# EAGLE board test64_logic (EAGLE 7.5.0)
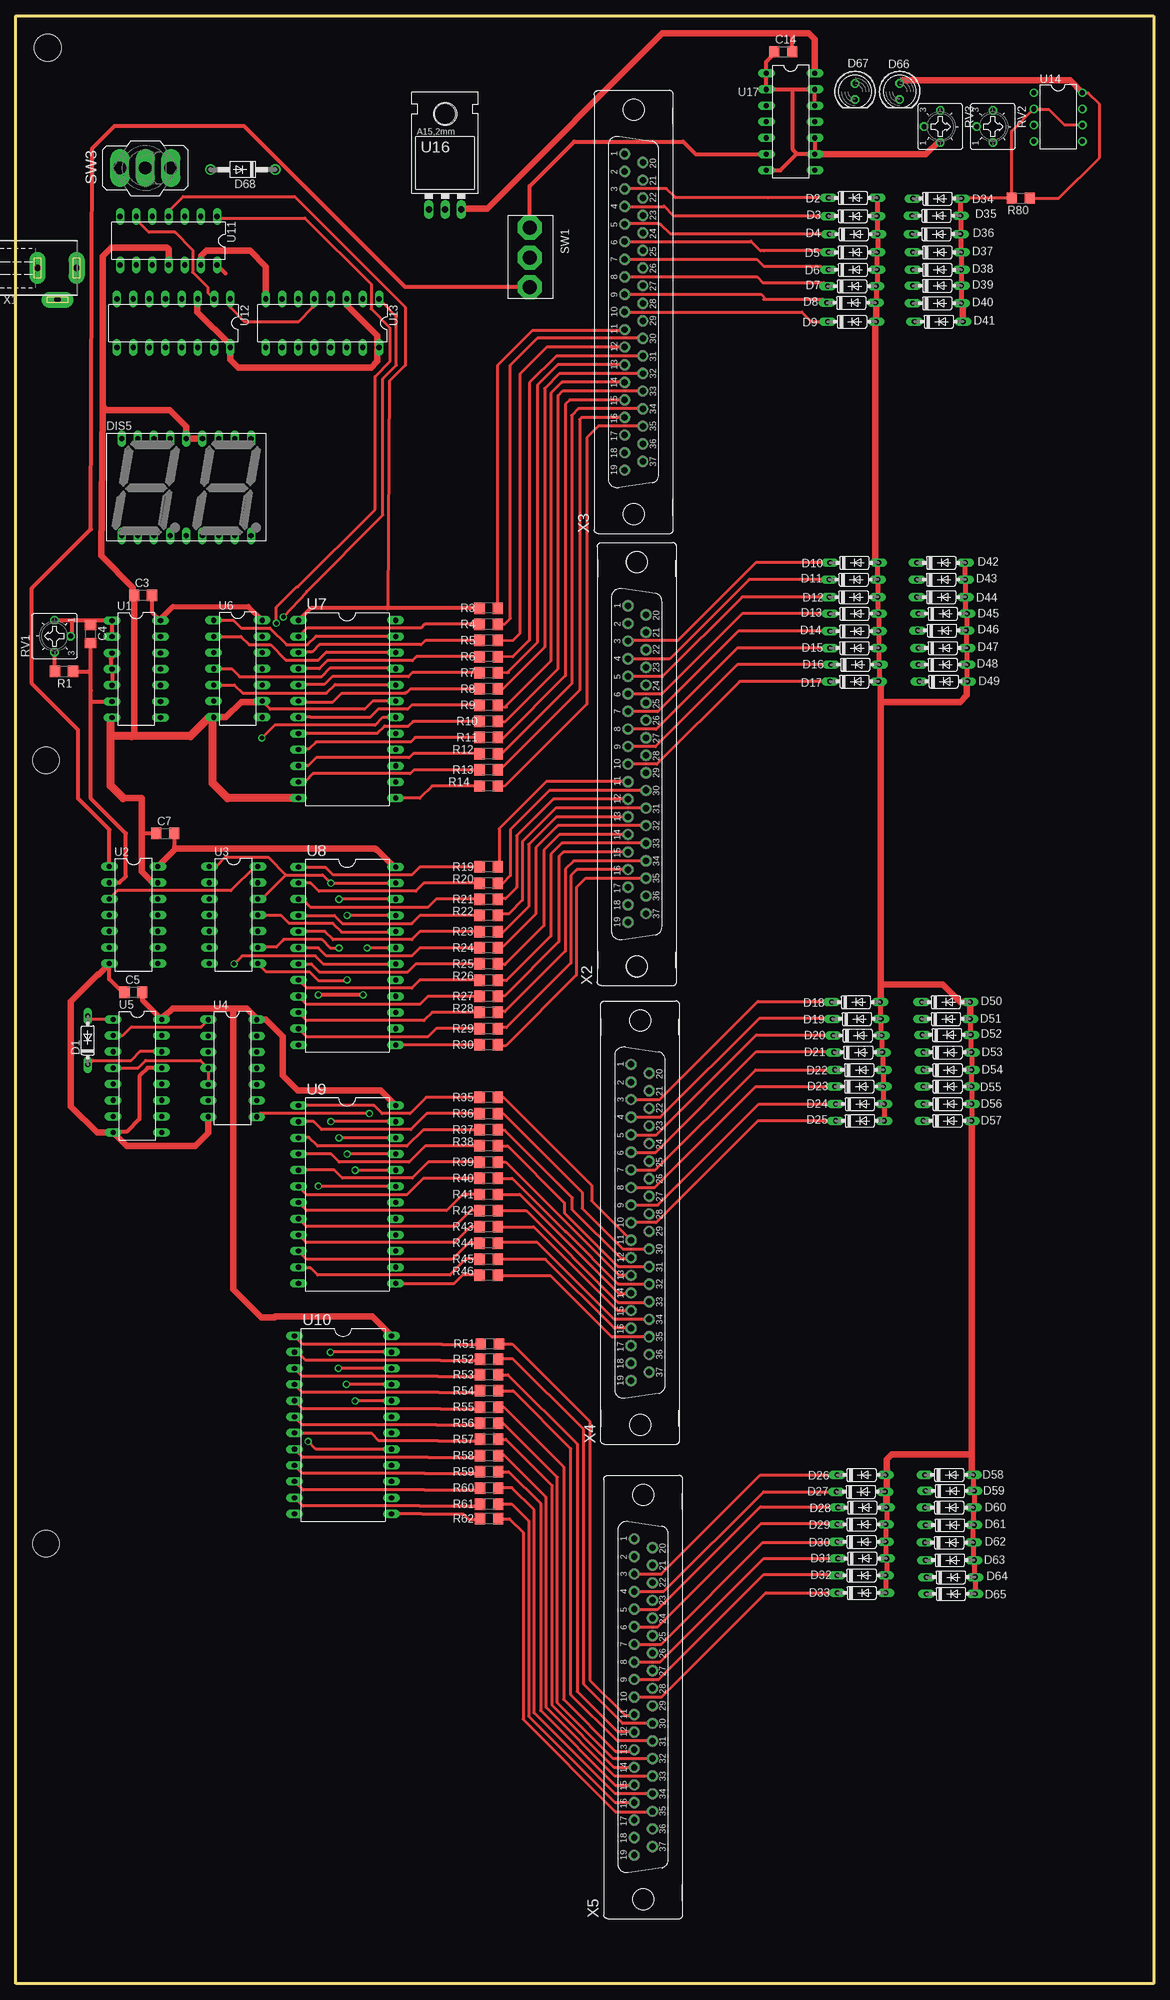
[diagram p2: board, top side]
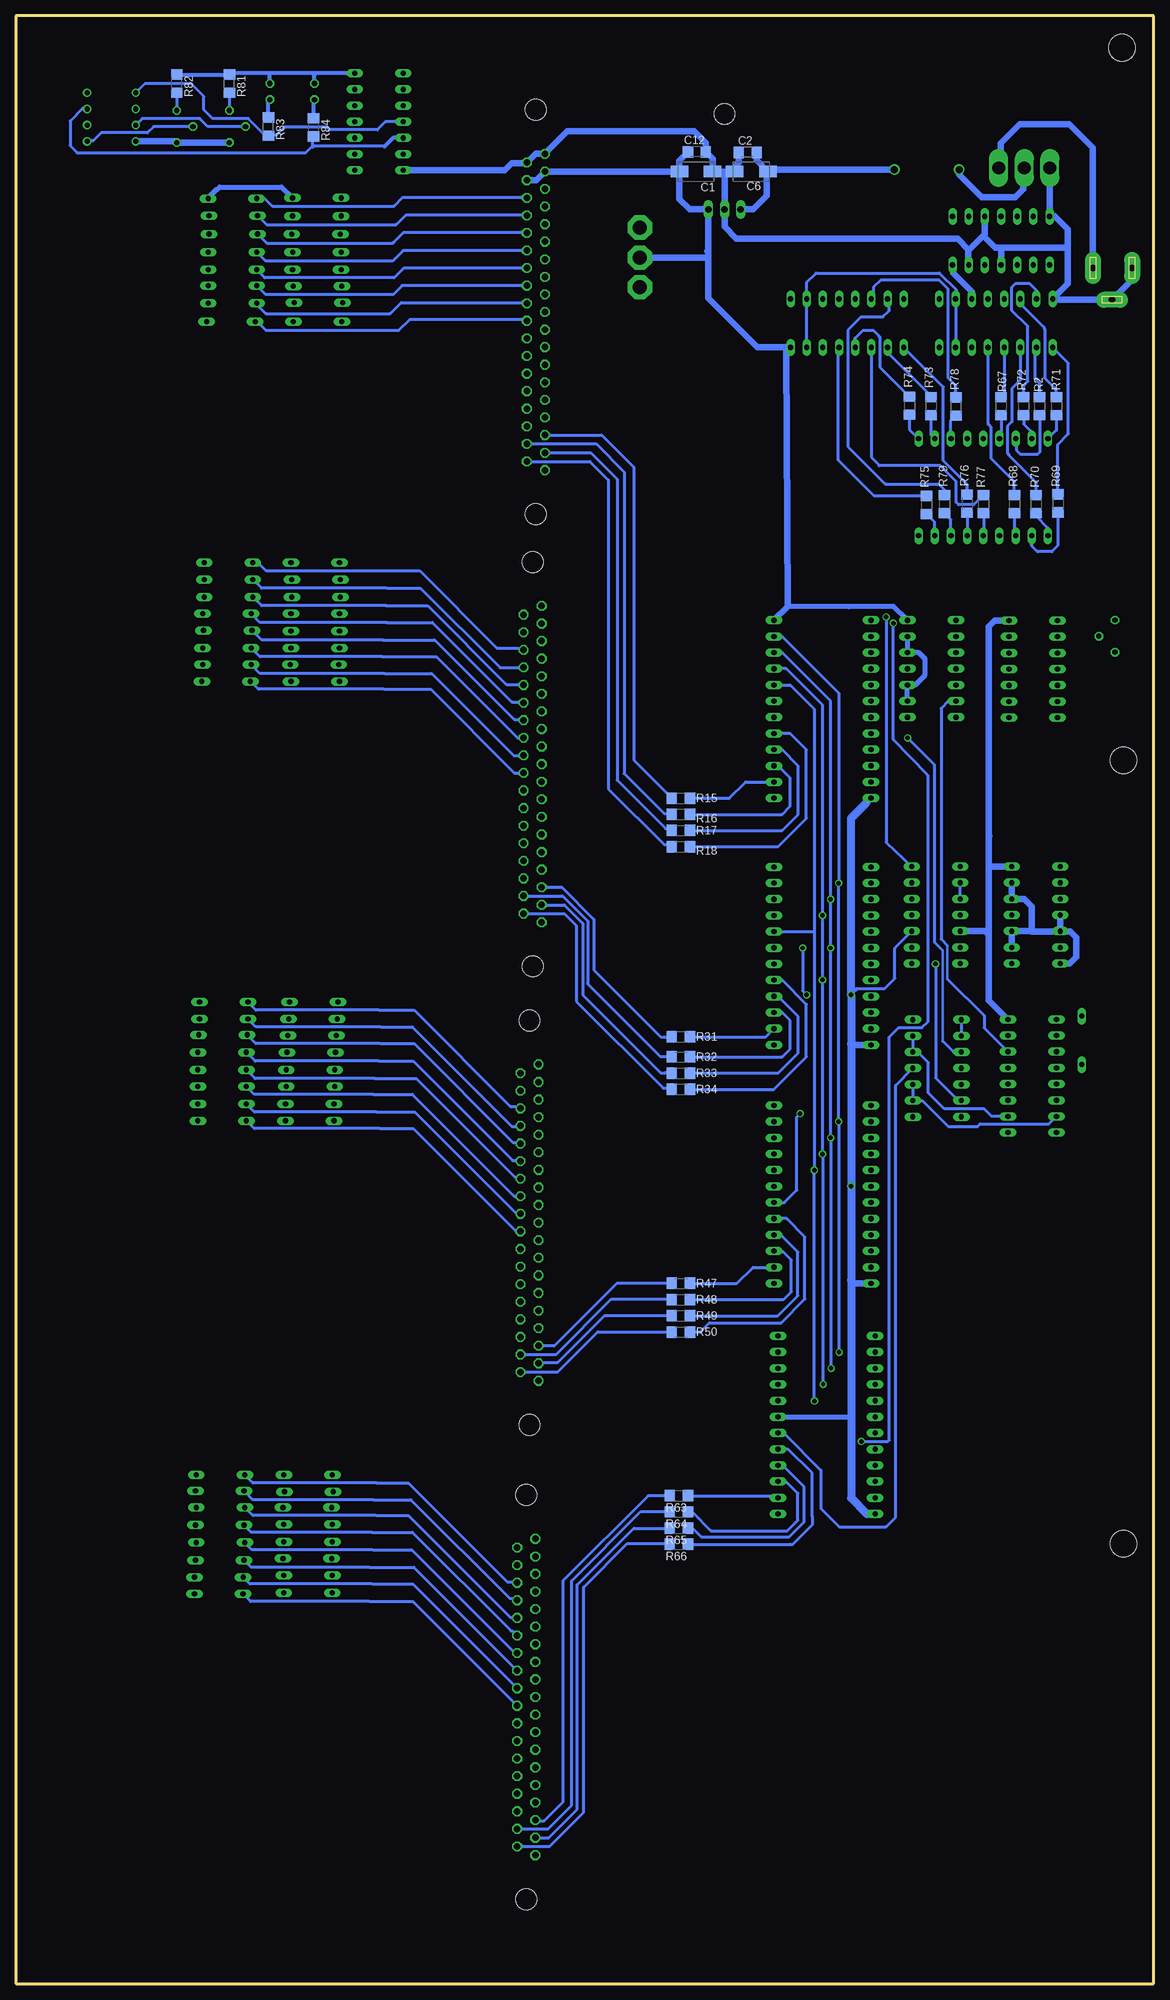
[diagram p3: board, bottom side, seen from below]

Size 178.62 x 309 mm. Coordinates in mm from the lower left corner, seen from the top.
Outline: 0,0 0,309 178.62,309 178.62,0 0,0
Copper layers (1*16): Top 0.035mm / dielectric 1.5mm / Bottom 0.035mm
Design rules "default *": minimum track width 10mil, minimum drill 24mil, track to track 8mil, track to pad 8mil, pad to pad 8mil, via to via 8mil, smd to smd 8mil, copper to edge 40mil, drill to drill 8mil, minimum pad ring 10mil, minimum via ring 8mil, stop-mask expansion 4mil, vias tented up to drill 0mil, thermal gap 10mil
Holes 4.2 mm at 5,304 4.75,69.12 4.75,192.12

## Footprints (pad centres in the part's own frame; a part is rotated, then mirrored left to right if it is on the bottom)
C/6032-28W = smd 2.75 x 1.8: + 2.625,0; - -2.625,0
C1206 = smd 1.6 x 1.8: 1 -1.4,0; 2 1.4,0
DO35-7 = drill 0.813 long: A 3.81,0; C -3.81,0
LED5MM = drill 0.813 octagon: A -1.27,0; K 1.27,0
DO41-10 = drill 1.118: A 5.08,0; C -5.08,0
HDSP-R = drill 0.813 long: 1 -10.16,-7.62; 2 -7.62,-7.62; 3 -5.08,-7.62; 4 -2.54,-7.62; 5 0,-7.62; 6 2.54,-7.62; 7 5.08,-7.62; 8 7.62,-7.62; 9 10.16,-7.62; 10 10.16,7.62; 11 7.62,7.62; 12 5.08,7.62; 13 2.54,7.62; 14 0,7.62; 15 -2.54,7.62; 16 -5.08,7.62; 17 -7.62,7.62; 18 -10.16,7.62
R1206 = smd 1.6 x 1.803: 1 -1.422,0; 2 1.422,0
CT6 = drill 0.813 octagon: A 2.515,0; E -2.515,0; S 0,-2.54
9077-1 = drill 2.2 pad 3.81 octagon: 1 4.7,-0.116; 2 0.06,-0.116; 3 -4.66,-0.116
320-916 = drill 2.007 long: 1 0,4.013; 2 0,0; 3 0,-4.013
DIL14 = drill 0.813 long: 1 -7.62,-3.81; 2 -5.08,-3.81; 3 -2.54,-3.81; 4 0,-3.81; 5 2.54,-3.81; 6 5.08,-3.81; 7 7.62,-3.81; 8 7.62,3.81; 9 5.08,3.81; 10 2.54,3.81; 11 0,3.81; 12 -2.54,3.81; 13 -5.08,3.81; 14 -7.62,3.81
DIL16 = drill 0.813 long: 1 -8.89,-3.81; 2 -6.35,-3.81; 3 -3.81,-3.81; 4 -1.27,-3.81; 5 1.27,-3.81; 6 3.81,-3.81; 7 6.35,-3.81; 8 8.89,-3.81; 9 8.89,3.81; 10 6.35,3.81; 11 3.81,3.81; 12 1.27,3.81; 13 -1.27,3.81; 14 -3.81,3.81; 15 -6.35,3.81; 16 -8.89,3.81
DIL24-6 = drill 0.813 long: 1 -13.97,-7.62; 2 -11.43,-7.62; 3 -8.89,-7.62; 4 -6.35,-7.62; 5 -3.81,-7.62; 6 -1.27,-7.62; 7 1.27,-7.62; 8 3.81,-7.62; 9 6.35,-7.62; 10 8.89,-7.62; 11 11.43,-7.62; 12 13.97,-7.62; 13 13.97,7.62; 14 11.43,7.62; 15 8.89,7.62; 16 6.35,7.62; 17 3.81,7.62; 18 1.27,7.62; 19 -1.27,7.62; 20 -3.81,7.62; 21 -6.35,7.62; 22 -8.89,7.62; 23 -11.43,7.62; 24 -13.97,7.62
DIL08 = drill 0.813 pad 1.27: 1 -3.81,-3.81; 2 -1.27,-3.81; 3 1.27,-3.81; 4 3.81,-3.81; 5 3.81,3.81; 6 1.27,3.81; 7 -1.27,3.81; 8 -3.81,3.81
78XXL = drill 1.016 long: GND 0,-3.81; IN -2.54,-3.81; OUT 2.54,-3.81 | hole 3.302: 0,11.176
733980-62 = drill 1 pad 2.5 long: 1 0,8.57; 2 0,2.42; 3 5,5.57
F37V = drill 1.016 octagon: 1 24.841,1.422; 2 22.073,1.422; 3 19.329,1.422; 4 16.561,1.422; 5 13.792,1.422; 6 11.049,1.422; 7 8.28,1.422; 8 5.512,1.422; 9 2.769,1.422; 10 0,1.422; 11 -2.769,1.422; 12 -5.512,1.422; 13 -8.28,1.422; 14 -11.049,1.422; 15 -13.818,1.422; 16 -16.561,1.422; 17 -19.329,1.422; 18 -22.098,1.422; 19 -24.841,1.422; 20 23.47,-1.422; 21 20.701,-1.422; 22 17.932,-1.422; 23 15.189,-1.422; 24 12.421,-1.422; 25 9.652,-1.422; 26 6.909,-1.422; 27 4.14,-1.422; 28 1.372,-1.422; 29 -1.372,-1.422; 30 -4.14,-1.422; 31 -6.909,-1.422; 32 -9.677,-1.422; 33 -12.421,-1.422; 34 -15.189,-1.422; 35 -17.958,-1.422; 36 -20.701,-1.422; 37 -23.47,-1.422 | hole 3.302: 31.75,0; -31.75,0

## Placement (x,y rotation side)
C1  [C/6032-28W]  71.86,284.54 180 bottom
C2  [C1206]  63.73,287.56 180 bottom
C3  [C1206]  19.95,218.03 0 top
C4  [C1206]  11.68,211.92 270 top
C5  [C1206]  18.45,155.7 0 top
C6  [C/6032-28W]  63.18,284.54 0 bottom
C7  [C1206]  23.45,180.62 0 top
C12  [C1206]  71.7,287.64 180 bottom
C14  [C1206]  120.48,303.38 0 top
D1  1N4148DO35-7  [DO35-7]  11.29,148.12 90 top
D2  1N4148DO35-7  [DO35-7]  131.38,280.43 0 top
D3  1N4148DO35-7  [DO35-7]  131.38,277.57 0 top
D4  1N4148DO35-7  [DO35-7]  131.51,274.73 0 top
D5  1N4148DO35-7  [DO35-7]  131.38,271.88 0 top
D6  1N4148DO35-7  [DO35-7]  131.38,269.15 0 top
D7  1N4148DO35-7  [DO35-7]  131.26,266.55 0 top
D8  1N4148DO35-7  [DO35-7]  131.13,263.95 0 top
D9  1N4148DO35-7  [DO35-7]  131.26,260.98 0 top
D10  1N4148DO35-7  [DO35-7]  131.62,223.12 0 top
D11  1N4148DO35-7  [DO35-7]  131.5,220.5 0 top
D12  1N4148DO35-7  [DO35-7]  131.5,217.75 0 top
D13  1N4148DO35-7  [DO35-7]  131.62,215.12 0 top
D14  1N4148DO35-7  [DO35-7]  131.62,212.38 0 top
D15  1N4148DO35-7  [DO35-7]  131.62,209.75 0 top
D16  1N4148DO35-7  [DO35-7]  131.75,207.12 0 top
D17  1N4148DO35-7  [DO35-7]  131.62,204.5 0 top
D18  1N4148DO35-7  [DO35-7]  131.88,154.12 0 top
D19  1N4148DO35-7  [DO35-7]  132,151.5 0 top
D20  1N4148DO35-7  [DO35-7]  132.12,148.88 0 top
D21  1N4148DO35-7  [DO35-7]  132.25,146.25 0 top
D22  1N4148DO35-7  [DO35-7]  132.38,143.5 0 top
D23  1N4148DO35-7  [DO35-7]  132.38,140.88 0 top
D24  1N4148DO35-7  [DO35-7]  132.5,138.12 0 top
D25  1N4148DO35-7  [DO35-7]  132.5,135.5 0 top
D26  1N4148DO35-7  [DO35-7]  132.75,79.88 0 top
D27  1N4148DO35-7  [DO35-7]  132.64,77.25 0 top
D28  1N4148DO35-7  [DO35-7]  132.88,74.75 0 top
D29  1N4148DO35-7  [DO35-7]  132.75,72.12 0 top
D30  1N4148DO35-7  [DO35-7]  132.75,69.38 0 top
D31  1N4148DO35-7  [DO35-7]  132.88,66.75 0 top
D32  1N4148DO35-7  [DO35-7]  132.75,64.12 0 top
D33  1N4148DO35-7  [DO35-7]  132.76,61.35 0 top
D34  1N4148DO35-7  [DO35-7]  144.64,280.32 0 top
D35  1N4148DO35-7  [DO35-7]  144.5,277.62 0 top
D36  1N4148DO35-7  [DO35-7]  144.5,274.75 0 top
D37  1N4148DO35-7  [DO35-7]  144.62,271.88 0 top
D38  1N4148DO35-7  [DO35-7]  144.62,269.12 0 top
D39  1N4148DO35-7  [DO35-7]  144.62,266.62 0 top
D40  1N4148DO35-7  [DO35-7]  144.62,263.88 0 top
D41  1N4148DO35-7  [DO35-7]  144.88,261 0 top
D42  1N4148DO35-7  [DO35-7]  145.25,223.12 0 top
D43  1N4148DO35-7  [DO35-7]  145.25,220.5 0 top
D44  1N4148DO35-7  [DO35-7]  145.25,217.75 0 top
D45  1N4148DO35-7  [DO35-7]  145.5,215.12 0 top
D46  1N4148DO35-7  [DO35-7]  145.38,212.5 0 top
D47  1N4148DO35-7  [DO35-7]  145.5,209.75 0 top
D48  1N4148DO35-7  [DO35-7]  145.5,207.12 0 top
D49  1N4148DO35-7  [DO35-7]  145.62,204.5 0 top
D50  1N4148DO35-7  [DO35-7]  146,154.12 0 top
D51  1N4148DO35-7  [DO35-7]  146,151.5 0 top
D52  1N4148DO35-7  [DO35-7]  146.12,149 0 top
D53  1N4148DO35-7  [DO35-7]  146.25,146.25 0 top
D54  1N4148DO35-7  [DO35-7]  146.25,143.5 0 top
D55  1N4148DO35-7  [DO35-7]  146.25,140.88 0 top
D56  1N4148DO35-7  [DO35-7]  146.25,138.12 0 top
D57  1N4148DO35-7  [DO35-7]  146.25,135.5 0 top
D58  1N4148DO35-7  [DO35-7]  146.5,79.88 0 top
D59  1N4148DO35-7  [DO35-7]  146.62,77.38 0 top
D60  1N4148DO35-7  [DO35-7]  146.5,74.75 0 top
D61  1N4148DO35-7  [DO35-7]  146.62,72 0 top
D62  1N4148DO35-7  [DO35-7]  146.5,69.25 0 top
D63  1N4148DO35-7  [DO35-7]  146.62,66.5 0 top
D64  1N4148DO35-7  [DO35-7]  146.76,63.83 0 top
D65  1N4148DO35-7  [DO35-7]  146.78,61.2 0 top
D66  [LED5MM]  138.75,297.12 270 top
D67  [LED5MM]  131.75,297.12 270 top
D68  1N4004  [DO41-10]  35.62,284.88 180 top
DIS5  HD-K123  [HDSP-R]  26.75,235 0 top
R1  [R1206]  7.54,206.06 180 top
R2  [R1206]  17.91,247.71 90 bottom
R3  [R1206]  74.22,216 0 top
R4  [R1206]  74.22,213.46 0 top
R5  [R1206]  74.22,210.92 0 top
R6  [R1206]  74.22,208.38 0 top
R7  [R1206]  74.22,205.84 0 top
R8  [R1206]  74.22,203.3 0 top
R9  [R1206]  74.22,200.76 0 top
R10  [R1206]  74.22,198.22 0 top
R11  [R1206]  74.22,195.68 0 top
R12  [R1206]  74.22,193.14 0 top
R13  [R1206]  74.22,190.6 0 top
R14  [R1206]  74.22,188.06 0 top
R15  [R1206]  74.22,186.16 180 bottom
R16  [R1206]  74.22,183.62 180 bottom
R17  [R1206]  74.22,181.07 180 bottom
R18  [R1206]  74.22,178.53 180 bottom
R19  [R1206]  74.22,175.36 0 top
R20  [R1206]  74.22,172.82 0 top
R21  [R1206]  74.22,170.28 0 top
R22  [R1206]  74.22,167.74 0 top
R23  [R1206]  74.22,165.2 0 top
R24  [R1206]  74.22,162.66 0 top
R25  [R1206]  74.22,160.12 0 top
R26  [R1206]  74.22,157.58 0 top
R27  [R1206]  74.22,155.04 0 top
R28  [R1206]  74.22,152.5 0 top
R29  [R1206]  74.22,149.96 0 top
R30  [R1206]  74.22,147.42 0 top
R31  [R1206]  74.22,148.69 180 bottom
R32  [R1206]  74.22,145.51 180 bottom
R33  [R1206]  74.22,142.97 180 bottom
R34  [R1206]  74.22,140.44 180 bottom
R35  [R1206]  74.22,139.17 0 top
R36  [R1206]  74.22,136.62 0 top
R37  [R1206]  74.22,134.08 0 top
R38  [R1206]  74.22,131.55 0 top
R39  [R1206]  74.22,129 0 top
R40  [R1206]  74.22,126.47 0 top
R41  [R1206]  74.22,123.92 0 top
R42  [R1206]  74.22,121.39 0 top
R43  [R1206]  74.22,118.84 0 top
R44  [R1206]  74.22,116.31 0 top
R45  [R1206]  74.22,113.77 0 top
R46  [R1206]  74.22,111.22 0 top
R47  [R1206]  74.22,109.95 180 bottom
R48  [R1206]  74.22,107.41 180 bottom
R49  [R1206]  74.22,104.88 180 bottom
R50  [R1206]  74.22,102.34 180 bottom
R51  [R1206]  74.41,100.45 0 top
R52  [R1206]  74.28,98.04 0 top
R53  [R1206]  74.28,95.62 0 top
R54  [R1206]  74.28,93.08 0 top
R55  [R1206]  74.28,90.54 0 top
R56  [R1206]  74.28,88 0 top
R57  [R1206]  74.28,85.46 0 top
R58  [R1206]  74.28,82.92 0 top
R59  [R1206]  74.28,80.38 0 top
R60  [R1206]  74.28,77.84 0 top
R61  [R1206]  74.28,75.3 0 top
R62  [R1206]  74.28,73.01 0 top
R63  [R1206]  74.53,76.62 180 bottom
R64  [R1206]  74.53,74.08 180 bottom
R65  [R1206]  74.53,71.54 180 bottom
R66  [R1206]  74.53,69 180 bottom
R67  [R1206]  23.95,247.71 90 bottom
R68  [R1206]  21.88,232.33 90 bottom
R69  [R1206]  15.04,232.46 90 bottom
R70  [R1206]  18.46,232.33 90 bottom
R71  [R1206]  15.26,247.71 90 bottom
R72  [R1206]  20.43,247.71 90 bottom
R73  [R1206]  34.98,247.71 90 bottom
R74  [R1206]  38.35,247.78 90 bottom
R75  [R1206]  35.65,232.21 90 bottom
R76  [R1206]  29.27,232.41 90 bottom
R77  [R1206]  26.69,232.33 90 bottom
R78  [R1206]  31.07,247.66 90 bottom
R79  [R1206]  32.86,232.33 90 bottom
R80  [R1206]  157.75,280.38 180 top
R81  [R1206]  145.12,298.38 270 bottom
R82  [R1206]  153.38,298.38 270 bottom
R83  [R1206]  139,291.62 270 bottom
R84  [R1206]  131.88,291.5 270 bottom
RV1  [CT6]  6.07,211.6 90 top
RV2  [CT6]  153.38,291.62 270 top
RV3  [CT6]  145.12,291.62 270 top
SW1  9077-1  [9077-1]  80.78,271.11 270 top
SW3  [320-916]  20.32,285.12 90 top
U1  74AC00N  [DIL14]  18.89,206.43 270 top
U2  74AC08N  [DIL14]  18.47,167.8 270 top
U3  74HC93N  [DIL14]  34.17,167.8 270 top
U4  74AC00N  [DIL14]  34,143.75 270 top
U5  4017N  [DIL16]  19.07,142.53 270 top
U6  7413N  [DIL14]  34.84,206.47 270 top
U7  74HC154N  [DIL24-6]  51.99,200.12 270 top
U8  74HC154N  [DIL24-6]  51.99,161.39 270 top
U9  74HC154N  [DIL24-6]  51.99,123.92 270 top
U10  74HC154N  [DIL24-6]  51.35,87.73 270 top
U11  74AC74N  [DIL14]  23.96,273.7 180 top
U12  4026N  [DIL16]  24.75,260.75 180 top
U13  4026N  [DIL16]  48.12,260.75 180 top
U14  LM393N  [DIL08]  163.62,293.12 270 top
U16  [78XXL]  67.38,282.43 0 top
U17  74AC08N  [DIL14]  121.62,292.38 270 top
X1  [733980-62]  0.95,269.43 270 top
X2  [F37V]  97.5,191.5 90 top
X3  [F37V]  97,262.5 90 top
X4  [F37V]  98,119.5 90 top
X5  [F37V]  98.5,45 90 top

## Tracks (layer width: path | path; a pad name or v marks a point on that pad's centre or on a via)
1
  Top 0.5: 118.1,280.43 103.58,280.43 102.12,281.88 95.62,281.88 X3.3
  Top 0.506: D2.C 118.1,280.43
2
  Bottom 0.5: 119.34,279.12 119.25,279.12 117.88,280.5 98.49,280.5 X3.22
  Bottom 0.506: D34.C 139.57,280.32 138.38,279.12 119.34,279.12
3
  Top 0.5: 120.08,277.57 103.3,277.57 101.75,279.12 101.69,279.06 X3.4
  Top 0.506: D3.C 120.08,277.57
4
  Bottom 0.5: 119,276.25 118.88,276.25 117.38,277.75 98.48,277.75 X3.23
  Bottom 0.506: D35.C 140.62,277.62 139.25,276.25 119,276.25
5
  Top 0.5: 117.48,274.73 102.78,274.73 101.25,276.25 101.12,276.25 101,276.38 95.66,276.38 X3.5
  Top 0.506: D4.C 117.48,274.73
6
  Bottom 0.5: 119.3,273.46 117.75,275 98.5,275 X3.24
  Bottom 0.506: 119.3,273.46 119.5,273.25 139.19,273.25 D36.C
7
  Top 0.5: 117.42,272.12 116.88,272.12 115.38,273.62 115.3,273.55 X3.6
  Top 0.506: D5.C 126.62,271.88 126.38,272.12 117.42,272.12
8
  Bottom 0.5: X3.25 117.85,272.15 119.08,270.91
  Bottom 0.506: 119.08,270.91 119.5,270.5 139.44,270.5 D37.C
9
  Top 0.5: X3.7 116.3,270.78 117.46,269.62
  Top 0.506: D6.C 126.85,269.15 126.38,269.62 117.46,269.62
10
  Bottom 0.5: X3.26 117.72,269.41 118.75,268.38
  Bottom 0.506: 118.75,268.38 119.25,267.88 139.56,267.88 D38.C
11
  Top 0.5: X3.8 116.36,268.01 117.25,267.12
  Top 0.506: 117.25,267.12 126.87,267.12 D7.C
12
  Bottom 0.5: X3.27 117.98,266.64 118.79,265.84
  Bottom 0.506: 118.79,265.84 119.38,265.25 139.44,265.25 D39.C
13
  Top 0.5: X3.9 116.98,265.27 117.75,264.5
  Top 0.506: 117.38,264.5 117.75,264.5 126.77,264.5 D8.C
14
  Bottom 0.5: D40.C 140.81,263.69 139.38,262.25 119.88,262.25 118.12,264 98.55,264 X3.28
15
  Top 0.5: X3.10 123.38,262.5 124.88,261 127.42,261 D9.C
16
  Bottom 0.5: D41.C 140.75,261 139.38,259.62 118.5,259.62 116.75,261.38 98.67,261.38 X3.29
17
  Top 0.5: D10.C 116.12,223.12 103.88,210.88 96.12,210.88 X2.3
18
  Bottom 0.5: D42.C 140.62,223.12 139.38,221.88 115.25,221.88 103.12,209.75 99.24,209.75 X2.22
19
  Top 0.5: D11.C 115.12,220.5 102.62,208 96.14,208 X2.4
20
  Bottom 0.5: 120.38,219.12 115.12,219.12 102.62,206.62 98.99,206.62 X2.23
  Bottom 0.506: 120.38,219.12 140.06,219.12 D43.C
21
  Top 0.5: D12.C 114,217.75 101.5,205.25 96.12,205.25 X2.5
22
  Bottom 0.5: 120.5,216.38 114,216.38 101.62,204 99,204 X2.24
  Bottom 0.506: 120.5,216.38 140.06,216.38 D44.C
23
  Top 0.5: D13.C 114,215.12 101.38,202.5 96.13,202.5 X2.6
24
  Bottom 0.5: 120.38,213.75 113.25,213.75 100.75,201.25 99.02,201.25 X2.25
  Bottom 0.506: 120.38,213.75 140.31,213.75 D45.C
25
  Top 0.5: D14.C 113.38,212.38 100.75,199.75 96.11,199.75 X2.7
26
  Bottom 0.5: 121,211 112.88,211 100.38,198.5 99.01,198.5 X2.26
  Bottom 0.506: 121,211 140.06,211 D46.C
27
  Top 0.5: D15.C 113.25,209.75 100.5,197 X2.8
28
  Bottom 0.5: 121.12,208.38 112.62,208.38 99.88,195.62 98.94,195.62 X2.27
  Bottom 0.506: 121.12,208.38 140.31,208.38 D47.C
29
  Top 0.5: D16.C 113.25,207.12 100.38,194.25 96.1,194.25 X2.9
30
  Bottom 0.5: 120.75,205.75 113.38,205.75 100.5,192.88 X2.28
  Bottom 0.506: 120.75,205.75 140.31,205.75 D48.C
31
  Top 0.5: D17.C 113.62,204.5 100.62,191.5 X2.10
32
  Bottom 0.5: 120.88,203.25 113.5,203.25 100.38,190.12 X2.29
  Bottom 0.506: 120.88,203.25 140.56,203.25 D49.C
33
  Top 0.5: X4.3 101.08,138.83 116.5,154.25 127.94,154.25 D18.C
34
  Bottom 0.5: 121.62,152.88 116.12,152.88 101,137.75 99.74,137.75 X4.22
  Bottom 0.506: 121.62,152.88 140.94,152.88 D50.C
35
  Top 0.5: X4.4 101.19,136.06 116.75,151.62 128.06,151.62 D19.C
  Top 0.506: 127.25,151.38 128.06,151.38 D19.C
36
  Bottom 0.5: 121.38,150.25 116.38,150.25 100.75,134.62 99.49,134.62 X4.23
  Bottom 0.506: 121.38,150.25 140.94,150.25 D51.C
37
  Top 0.5: X4.5 100.54,133.29 116.25,149 127.5,149
  Top 0.506: 127.5,149 128.19,149 D20.C
38
  Bottom 0.5: 121.5,147.62 116.12,147.62 100.62,132.12 99.63,132.12 X4.24
  Bottom 0.506: 121.5,147.62 140.94,147.62 D52.C
39
  Top 0.5: X4.6 100.42,130.55 116.25,146.38 127.75,146.38 127.88,146.25
  Top 0.506: D21.C 127.88,146.25 127.62,146.25
40
  Bottom 0.5: 121.62,144.88 116.25,144.88 100.62,129.25 99.52,129.25 X4.25
  Bottom 0.506: 121.62,144.88 141.06,144.88 D53.C
41
  Top 0.5: X4.7 100.41,127.78 116.12,143.5 D22.C
42
  Bottom 0.5: 122.25,142.12 115.75,142.12 100.25,126.62 99.64,126.62 X4.26
  Bottom 0.506: 122.25,142.12 141.06,142.12 D54.C
43
  Top 0.5: X4.8 100.26,125.01 116.12,140.88 D23.C
44
  Bottom 0.5: 122.5,139.62 116.38,139.62 100.38,123.62 99.44,123.62 X4.27
  Bottom 0.506: 122.5,139.62 141.19,139.62 D55.C
45
  Top 0.5: X4.9 100.77,122.27 116.62,138.12 D24.C
46
  Bottom 0.5: 122,136.88 116,136.88 100.12,121 99.55,121 X4.28
  Bottom 0.506: 122,136.88 141.19,136.88 D56.C
47
  Top 0.5: D25.C 116.5,135.5 100.5,119.5 X4.10
48
  Bottom 0.5: 121.5,134.25 116.25,134.25 100,118 99.55,118 X4.29
  Bottom 0.506: 121.5,134.25 141.19,134.25 D57.C
49
  Top 0.5: X5.3 101.33,64.33 116.88,79.88 D26.C
50
  Bottom 0.5: 122,78.62 117,78.62 101.5,63.12 100.11,63.12 X5.22
  Bottom 0.506: 122,78.62 141.44,78.62 D58.C
51
  Top 0.5: X5.4 101.69,61.56 117.38,77.25 D27.C
52
  Bottom 0.5: 122.5,76 116.62,76 101.12,60.5 100.23,60.5 X5.23
  Bottom 0.506: 122.5,76 141.44,76 D59.C
53
  Top 0.5: X5.5 100.79,58.79 116.88,74.88 128.94,74.88 D28.C
54
  Bottom 0.5: 122.12,73.5 117,73.5 101,57.5 100,57.5 X5.24
  Bottom 0.506: 122.12,73.5 141.44,73.5 D60.C
55
  Top 0.5: X5.6 100.8,56.05 117,72.25 128.81,72.25 D29.C
56
  Bottom 0.5: 122.75,70.88 116.38,70.88 100.88,55.38 100.64,55.38 X5.25
  Bottom 0.506: 122.75,70.88 141.69,70.88 D61.C
57
  Top 0.5: X5.7 101.28,53.28 117.25,69.25 128.38,69.25 128.5,69.12 128.69,69.12 D30.C
58
  Bottom 0.5: 122.62,68.12 116.5,68.12 100.5,52.12 100.14,52.12 X5.26
  Bottom 0.506: 122.62,68.12 141.56,68.12 D62.C
59
  Top 0.5: X5.8 101.14,50.51 117.38,66.75 D31.C
60
  Bottom 0.5: 123.12,65.38 116.16,65.38 X5.27
  Bottom 0.506: 123.12,65.38 141.69,65.38 D63.C
61
  Top 0.5: X5.9 100.89,47.77 117.38,64.25 128.81,64.25 D32.C
62
  Bottom 0.5: 122.75,62.75 116.3,62.75 X5.28
  Bottom 0.506: 122.75,62.75 141.88,62.75 D64.C
63
  Top 0.5: X5.10 101.38,45 117.75,61.38 128.93,61.38 D33.C
64
  Bottom 0.5: 123.12,60 116.29,60 X5.29
  Bottom 0.506: 123.12,60 141.76,60 D65.C
+5V
  Top 0.5: R80.1 163.75,280.38 170.12,286.75 170.12,295.12 168.38,296.88 167.5,296.88 U14.8
  Top 0.51: 44.15,104.9 44,104.75
  Top 0.61: C7.2 24.86,178.5 25.11,178.25 | 32.88,268.59 U11.14 | C3.2 21.36,215.4 U1.14 | C14.2 121.88,305.75 122.38,306.25
  Top 0.813: U1.14 22.7,214.33 24.62,216.25 36.5,216.25 U6.14 | C5.2 19.86,154.44 U5.16
  Top 1.016: U2.14 25.11,178.25 56.38,178.25 56.5,178.12 56.62,178.12 59.39,175.36 U8.24 | U13.3 51.94,263.56 56.75,258.75 56.75,257.21 U13.16 56.75,256.68 56.75,254.75 55.75,253.75 34.88,253.75 33.64,254.99 U12.16 33.64,257.36 28.5,262.5 28.5,264.5 U12.3 | 33.88,153.12 36.25,153.12 37.81,151.56 U4.14 39.25,151.38 41.88,148.75 41.88,142.62 44.25,140.25 57.26,140.25 U9.24 | 33.88,153.12 24.59,153.12 23.38,151.92 | 33.88,153.12 34.12,152.88 34.12,109 38.5,104.62 40.62,104.62 40.75,104.75 44,104.75 55.92,104.75 U10.24 | U16.OUT 70.05,278.75 74,278.75 101.5,306.25 122.38,306.25 124.5,306.25 125.44,305.31 U17.14 | U14.8 165.5,298.88 139.23,298.88 D66.A
  Top 1.27: 23.38,151.92 U5.16
  Bottom 0.61: U17.14 132,300 | 132,300 138.62,300 | 138.62,300 144.93,300 R81.1 R82.1 | D66.A 138.75,299.87 138.62,300 | D67.A 131.75,299.75 132,300
  Bottom 0.813: U6.14 38.72,214.09 40.88,216.25 47.88,216.25 | 47.88,216.25 57.45,216.25 | 47.84,216.21 47.88,216.25
  Bottom 1.016: U12.3 28.56,265.69 31.5,268.62 31.5,269.81 U11.14 | U1.14 24.95,214.04 25.88,213.12 25.88,180.25 | 25.88,180.25 25.88,175.5 | 25.88,175.5 25.88,164.75 | 25.88,164.75 25.88,154.42 U5.16 | U2.14 25.8,175.42 25.88,175.5 | U3.5 26.39,165.26 25.88,164.75 | 25.8,180.18 25.88,180.25 | C1.+ 74.48,286.26 C12.2 | 69.92,272.25 U16.OUT 72.87,278.62 74.5,280.25 C1.+ | 69.92,272.25 69.92,271 | 69.92,271 69.92,264.66 62.25,257 57.08,257 U13.16 57.7,256.25 57.45,216.25 U7.24 | 70.11,272.05 69.92,272.25 | SW1.2 69.97,271.05 69.92,271 | C1.+ 74.51,284.57 X3.2 96.95,283.2 X3.21
A  (via drill 0.7)
  Top 0.5: v49.45,172.82 U8.23 | U9.23 v49.45,135.36 | U3.1 31.42,175.42 32.88,176.88 39.62,176.88 42.38,174.12
  Top 0.506: U6.1 34.16,214.09 35.38,212.88 39.88,212.88 42.5,210.25 45.75,210.25 47.12,211.62 59.54,211.62 U7.23 | v49.45,172.82 48.15,174.12 42.38,174.12 38.59,170.34 U3.12 | U10.23 49.41,99.16 v49.38,99.12
  Bottom 0.5: U7.23 58.34,211.56 49.45,202.66 v49.45,172.82 v49.45,135.36
  Bottom 0.506: v49.38,99.12 49.38,135.28 v49.45,135.36
A1
  Bottom 0.5: R2.1 17.91,240.47 18.25,240.12 20.88,240.12 21.5,240.75 21.5,242.45 DIS5.16
A2
  Bottom 0.5: R73.1 34.98,243.22 DIS5.11
B  (via drill 0.7)
  Top 0.5: U8.22 v50.72,170.28 | U9.22 v50.72,132.81
  Top 0.506: U6.2 35.32,211.56 36.62,210.25 40,210.25 42.38,207.88 47.5,207.88 48.75,209.12 59.5,209.12 U7.22 | v50.72,162.62 49.38,162.62 48,164 42,164 42,163.88 40.88,162.75 38.01,162.75 U3.9 | U10.22 v50.63,96.62 v50.62,96.62
  Bottom 0.5: U7.22 58.34,209.01 50.72,201.4 v50.72,170.28 50.72,164.88 | v50.72,132.81 v50.72,162.62
  Bottom 0.506: v50.72,162.62 50.72,164.88 | v50.62,96.62 50.62,132.72 v50.72,132.81
B1
  Bottom 0.5: R67.1 23.95,242.88 DIS5.15
B2
  Bottom 0.5: R74.1 38.35,244.06 DIS5.10
C  (via drill 0.7)
  Top 0.5: U8.21 v51.99,167.74 | U9.21 v51.99,130.28
  Top 0.506: U6.4 33.9,206.47 35.12,205.25 48,205.25 49.38,206.62 59.46,206.62 U7.21 59.59,206.5 | v51.99,157.62 51.87,157.5 47.5,157.5 46.12,158.88 39.28,158.88 U3.8 | U10.21 51.92,94.08 v51.88,94.12
  Bottom 0.5: U7.21 57.7,206.47 51.99,200.76 v51.99,167.74 51.99,160.75 | v51.99,130.28 v51.99,157.62 | 51.99,158.62 51.99,160
  Bottom 0.506: 51.99,160 51.99,160.75 | v51.99,157.62 51.99,158.62 | v51.88,94.12 51.88,130.16 v51.99,130.28
C1
  Bottom 0.5: R68.1 21.88,227.59 DIS5.3
C2
  Bottom 0.5: DIS5.8 34.37,229.51 R75.1
CL  (via drill 0.7)
  Top 0.5: U3.14 37.55,175.42 33.75,171.62 15.95,171.62 U2.3 | U13.1 57.02,264.49 59.75,261.75 59.75,254.12 57.62,252 57.62,230.62 45.62,218.62 45.62,218.5 v42,214.62
  Bottom 0.5: 37.17,175.42 U3.14 42,179.19 v42,214.62
D  (via drill 0.7)
  Top 0.5: v53.26,127.73 U9.20
  Top 0.506: U6.5 34.31,203.94 35.62,202.62 48.75,202.62 50.12,204 59.55,204 U7.20 | 59.56,165.25 U8.20 59.53,165.12 51.12,165.12 49.75,166.5 42.88,166.5 41.62,167.75 38.03,167.75 U3.11 | U10.20 53.29,91.54 v53.25,91.5
  Bottom 0.5: U7.20 57.07,203.94 53.26,200.12 53.26,165.2 | 53.26,165.2 v53.26,127.73 | U8.20 53.26,165.2
  Bottom 0.506: v53.25,91.5 v53.25,127.72 v53.26,127.73
D1
  Bottom 0.5: R69.1 15.04,225.83 16,224.88 18.25,224.88 19.12,225.75 DIS5.2
D2
  Bottom 0.5: R76.1 29.27,227.4 DIS5.6
E1
  Bottom 0.5: DIS5.1 16.59,228.59 18.46,230.47 R70.1
E2
  Bottom 0.5: R77.1 26.69,227.44 DIS5.5
F1
  Bottom 0.5: R71.1 15.26,243.95 DIS5.18
F2
  Bottom 0.5: DIS5.12 31.83,245.47 R78.1
G1
  Bottom 0.5: R72.1 20.43,244.93 19.25,243.75 19.25,242.74 DIS5.17
G2
  Bottom 0.5: DIS5.7 31.83,229.88 R79.1
GND  (via drill 0.7)
  Top 0.5: U7.19 56.02,201.4 54.75,200.12 39.92,200.12 U6.9 | U8.19 55.16,162.66 v55.12,162.62 | U9.19 47.55,125.19 v47.5,125.25
  Top 0.61: v54.5,155.25 v47.5,155.25 | C5.1 16.68,155.7 14.62,157.75 14.62,160.14 U2.7 | U5.13 20.68,143.8 19.38,142.5 19.38,135.75 17.38,133.75 15.37,133.75 U5.8 | C7.1 20.13,180.62 19.75,181 | 39.02,268.59 39.23,268.38 | C14.1 119.08,303.08 117.75,301.75 117.75,300.06 U17.1 U17.2 121.88,297.46 | 121.88,297.46 U17.13 U17.12 | 122.62,287.38 122.7,287.29 U17.9 U17.10 | 122.62,287.38 122,288 122,297.33 121.88,297.46 | U17.7 120,284.75 122.62,287.38
  Top 1.016: U13.8 39.23,268.38 39.23,269.64 36.75,272.12 29.88,272.12 29.12,271.38 29.12,269.98 U11.13 | DIS5.13 DIS5.14 26.75,244.5 24.12,247.12 14.12,247.12 13.62,247.62 | U11.11 23.96,272.38 23.71,272.62 15,272.62 13.62,271.25 13.62,247.62 | 16.84,186.16 19.72,186.16 19.75,186.12 19.75,181 19.75,174.62 21.62,172.75 22.15,172.75 U2.13 | U6.7 32.98,198.85 35.38,201.25 38.51,201.25 U6.9 | 13.62,247.62 13.38,224.25 18.38,219.25 18.38,218.21 C3.1 18.55,196.31 18.12,195.88 | U2.7 12.98,158.5 12.88,158.5 8.62,154.25 8.62,137.75 12.73,133.64 U5.8 17.4,131.5 28.12,131.5 30.19,133.56 U4.7 | RV3.A 144.74,289.11 142.88,287.25 125.48,287.25 U17.9
  Top 1.27: 16.84,186.16 14.88,188.12 14.88,195.75 | 14.88,195.75 14.88,198.59 U1.7 | 14.88,195.75 15,195.88 18.12,195.88 27.38,195.88 30.36,198.85 U6.7 30.88,198.69 30.88,188.5 33.22,186.16 U7.12
  Bottom 0.5: v55.12,162.62 55.12,155.88 v54.5,155.25 | U3.10 40.62,162.62 40.62,157.88 42.25,156.25 46.75,156.25 46.75,156 v47.5,155.25
  Bottom 0.813: U6.9 U6.10 37.44,203.94 35.88,205.5 35.88,208 36.88,209 38.64,209 U6.12 U6.13 | 47.3,147.42 47.5,147.62 | 46.95,109.95 47.5,110.5 | U10.19 47.5,89
  Bottom 1.016: U11.3 26.5,274.75 26.75,274.5 | 26.75,274.5 29,272.25 | 29,272.25 29.12,272.12 29.12,269.98 U11.13 | 23.96,271.34 U11.11 23.96,272.46 24.12,272.62 | 13.5,272.38 13.5,275.5 15.51,277.51 U11.7 16.3,277.55 SW3.1 | 13.5,272.38 13.5,266.92 U12.8 15.73,264.43 X1.3 3.38,267.58 X1.2 | 24.12,272.62 13.75,272.62 13.5,272.38 | 24.12,272.62 24.88,272.62 26.75,274.5 | U2.13 U2.12 20.34,170.34 19.12,169.12 19.12,165.25 | 19.12,165.25 15.25,165.25 | 15.25,165.25 U2.5 13.12,165.25 12.12,164.25 12.12,161.25 13.2,160.18 U2.7 | 19.12,165.25 19.14,165.26 U2.10 U2.9 | U2.4 14.66,165.84 15.25,165.25 | 29,272.25 30.75,274 65.5,274 67.38,275.88 U16.GND 67.38,284.42 67.5,284.54 | C6.- 66.5,284.54 | 66.5,284.54 67.5,284.54 | 67.5,284.54 C1.- 69.23,286.56 C12.1 70.31,289.06 72.12,290.88 92.04,290.88 X3.1 97.05,287.34 X3.20 98.52,285.88 100.75,285.88 101.87,284.75 U17.7 | C2.2 65.12,285.92 66.5,284.54 | 45.2,185.32 U7.12 | U14.4 153.58,289.31 RV2.A RV3.A | 46.95,109.95 U9.12 | 47.3,147.42 U8.12 | 45.01,73.76 U10.12
  Bottom 1.27: 45.01,73.76 47.5,76.25 47.5,89 47.5,110.5 v47.5,125.25 47.5,147.62 v47.5,155.25 47.5,183.03 45.2,185.32
L1
  Top 0.5: R3.2 75.64,254.14 81.12,259.62 95.47,259.62 X3.11
L2
  Top 0.5: R4.2 76.71,213.46 77.62,214.38 77.62,254.12 81.86,258.36 X3.30
L3
  Top 0.406: 78.03,210.92 R5.2
  Top 0.5: X3.12 83.36,256.99 79.12,252.75 79.12,212.02 78.03,210.92
L4
  Top 0.406: R6.2 78.03,208.38
  Top 0.5: X3.31 84.84,255.59 80.62,251.38 80.62,210.98 78.03,208.38
L5
  Top 0.406: R7.2 77.12,205.84 77.39,205.84
  Top 0.5: X3.13 85.09,254.22 81.88,251 81.88,210.59 77.12,205.84
L6
  Top 0.406: R8.2 76.44,203.3
  Top 0.5: X3.32 85.32,252.82 83,250.5 83,209.86 76.44,203.3
L7
  Top 0.406: R9.2 75.95,200.44 76.75,200.44 77.07,200.44
  Top 0.5: X3.14 85.7,251.45 84,249.75 84,207.69 76.75,200.44
L8
  Top 0.406: R10.2 76.12,198.22
  Top 0.5: 76.12,198.22 76.84,198.22 85.12,206.5 85.12,249.38 85.88,250.12 98.38,250.12 X3.33
L9
  Top 0.406: R11.2 76.12,195.68 76.34,195.46
  Top 0.5: X3.15 86.93,248.68 86.25,248 86.25,205.38 76.34,195.46
L10
  Top 0.406: R12.2 75.64,192.99
  Top 0.5: X3.34 88.31,247.31 87.25,246.25 87.25,204.12 76.25,193.12 75.65,193.12 R12.2
L11
  Top 0.406: R13.2 76.12,190.6
  Top 0.5: X3.16 88.81,245.94 88.5,245.62 88.5,203.12 76.25,190.88 75.91,190.88 R13.2
L12
  Top 0.406: R14.2 76.75,188.06
  Top 0.5: X3.35 91.42,244.54 89.62,242.75 89.62,200.93 76.75,188.06
L13
  Bottom 0.5: X3.17 86.67,243.17 81.62,238.12 81.62,192.14 R15.2
L14
  Bottom 0.5: X3.36 87.55,241.8 83.12,237.38 83.12,190 76.88,183.75 75.25,183.75 75.12,183.62 75.63,183.62 R16.2
L15
  Bottom 0.5: X3.18 88.4,240.4 84.25,236.25 84.25,189 76.62,181.38 75.94,181.38 R17.2
L16
  Bottom 0.5: X3.37 88.53,239.03 85.62,236.12 85.62,187.62 76.88,178.88 75.98,178.88 R18.2
L17
  Top 0.5: X2.11 83.23,188.73 75.88,181.38 75.88,175.6 R19.2
L18
  Top 0.5: X2.30 83.73,187.36 77.62,181.25 77.62,174 76.25,172.62 75.83,172.62 R20.2
L19
  Top 0.5: X2.12 84.36,185.99 78.62,180.25 78.62,172.12 76.88,170.38 75.73,170.38 R21.2
L20
  Top 0.5: 75.64,167.89 R22.2 76.25,167.75 76.5,168 77.38,168 79.5,170.12 79.5,179.38 84.72,184.59 X2.31
L21
  Top 0.5: X2.13 84.84,183.22 80.5,178.88 80.5,169.12 76.5,165.12 75.71,165.12 R23.2
L22
  Top 0.5: X2.32 85.07,181.82 81.62,178.38 81.62,168 76.5,162.88 75.85,162.88 R24.2
L23
  Top 0.5: X2.14 85.33,180.45 82.88,178 82.88,166.12 76.75,160 75.76,160 R25.2
L24
  Top 0.5: X2.33 85.7,179.08 84,177.38 84,164.5 77,157.5 75.72,157.5 R26.2
L25
  Top 0.5: X2.15 85.93,177.68 85.25,177 85.25,163.62 76.75,155.12 75.72,155.12 R27.2
L26
  Top 0.5: X2.34 87.56,176.31 86.25,175 86.25,162.12 76.75,152.62 76.25,152.62 75.88,153 75.88,152.74 R28.2
L27
  Top 0.5: X2.16 88.06,174.94 87.12,174 87.12,160.25 77,150.12 75.8,150.12 R29.2
L28
  Top 0.5: X2.35 89.42,173.54 88,172.12 88,158.38 76.88,147.25 75.81,147.25 R30.2
L29
  Bottom 0.5: R31.2 77.39,148.69 87.88,159.18 87.88,167.12 92.92,172.17 X2.17
L30
  Bottom 0.5: R32.2 77.39,145.51 88.88,157 88.88,166.88 92.8,170.8 X2.36
L31
  Bottom 0.5: R33.2 76.75,142.97 76.78,143 77.38,143 89.62,155.25 89.62,166.5 92.53,169.4 X2.18
L32
  Bottom 0.5: 76.12,140.44 R34.2 75.83,140.62 77,140.62 90.62,154.25 90.62,166.12 92.53,168.03 X2.37
L33
  Top 0.5: X4.11 90.38,122.93 90.38,125.38 76.58,139.17 R35.2
L34
  Top 0.5: X4.30 99.41,115.38 95.25,115.38 88.88,121.75 88.88,124.25 76.5,136.62 R36.2
L35
  Top 0.5: X4.12 96.46,113.88 95,113.88 87.38,121.5 87.38,123.38 76.75,134 75.72,134 R37.2
L36
  Top 0.5: X4.31 99.39,112.62 94.5,112.62 86.12,121 86.12,122.62 77.2,131.55 R38.2
L37
  Top 0.5: X4.13 96.55,111.25 94.62,111.25 76.87,129 R39.2
L38
  Top 0.5: X4.32 99.37,109.88 94.5,109.88 86.38,118 86.25,118.12 77.91,126.47 R40.2
L39
  Top 0.5: X4.14 96.5,108.38 94.62,108.38 79.08,123.92 R41.2
L40
  Top 0.5: X4.33 99.34,107 94.5,107 80.11,121.39 R42.2
L41
  Top 0.5: X4.15 96.51,105.75 94.38,105.75 81.28,118.84 R43.2
L42
  Top 0.5: 76.12,116.31 R44.2 75.71,116.38 81.88,116.38 93.94,104.31 X4.34
L43
  Top 0.5: R45.2 76.25,113.77 | 76.25,113.77 76.44,113.77 | X4.16 93.94,102.94 83.12,113.75 76.27,113.75 76.25,113.77
L44
  Top 0.5: R46.2 76.44,111.22 76.54,111.12 84,111.12 93.58,101.54 X4.35
L45
  Bottom 0.5: 75.64,110.42 R47.2 84.3,109.95 94.12,100.12 96.53,100.12 X4.17
L46
  Bottom 0.5: X4.36 93.83,98.8 85.12,107.5 75.72,107.5 R48.2
L47
  Bottom 0.5: R49.2 86.25,104.88 93.62,97.5 96.48,97.5 X4.18
L48
  Bottom 0.5: 76.12,102.34 R50.2 75.68,102.38 87.25,102.38 93.59,96.03 X4.37
L49
  Top 0.5: R51.2 77.92,100.45 90.12,88.25 90.12,47.62 95.62,42.12 96.97,42.12 X5.11
L50
  Top 0.5: X5.30 95.27,40.86 89.12,47 89.12,87 78,98.12 75.79,98.12 R52.2
L51
  Top 0.5: X5.12 96.94,39.62 94.38,39.62 88.12,45.88 88.12,84.75 77.25,95.62 R53.2
L52
  Top 0.5: X5.31 94.41,38.09 87.12,45.38 87.12,84 78.04,93.08 R54.2 75.75,93.12
L53
  Top 0.5: X5.13 96.86,36.5 94.12,36.5 86,44.62 86,81.12 76.58,90.54 R55.2
L54
  Top 0.5: X5.32 93.8,35.32 85,44.12 85,79.5 76.5,88 R56.2
L55
  Top 0.5: X5.14 97.03,34 93.88,34 84.12,43.75 84.12,78.25 76.91,85.46 R57.2
L56
  Top 0.5: X5.33 94.05,32.58 83.25,43.38 83.25,76.38 76.62,83 75.78,83 R58.2
L57
  Top 0.5: X5.15 97.02,31.12 94.12,31.12 82.38,42.88 82.38,75.38 77.37,80.38 R59.2
L58
  Top 0.5: X5.34 94.06,29.81 81.38,42.5 81.38,74.38 77.88,77.88 75.74,77.88 R60.2
L59
  Top 0.5: R61.2 77.82,75.3 80.5,72.62 80.5,42 94,28.5 97.02,28.5 X5.16
L60
  Top 0.5: R62.2 77.49,73.01 79.62,70.88 79.62,41.5 94.12,27 99.88,27 X5.35
L61
  Bottom 0.5: R63.2 79.38,76.62 92.75,63.25 92.75,28.5 95.75,25.5 96.91,25.5 X5.17
L62
  Bottom 0.5: X5.36 95.08,24.3 91.38,28 91.38,63.25 80.5,74.12 76,74.12 R64.2
L63
  Bottom 0.5: X5.18 94.97,22.9 90.5,27.38 90.5,62.62 81.62,71.5 75.99,71.5 R65.2
L64
  Bottom 0.5: X5.37 94.84,21.53 89.5,26.88 89.5,62.25 82.62,69.12 76.08,69.12 R66.2
MR
  Bottom 0.5: U3.3 U3.2
N$1
  Top 0.61: U1.3 15.09,208.21 14.88,208 14.88,206.63 U1.4 U1.5
N$2
  Top 0.61: RV1.A 8.88,214.12 | 8.88,214.12 11.62,214.12 | 11.62,214.12 15.09,214.12 U1.1 U1.2 | RV1.S 8.88,211.6 8.88,214.12 | C4.1 11.62,213.32 11.62,214.12
N$3
  Top 0.5: 14.99,201.25 14.12,201.25
  Top 0.61: C4.2 11.68,205.75 | 11.68,205.75 11.68,203.19 11.75,203.12 11.75,201.38 | U1.6 14.99,201.25 11.88,201.25 11.75,201.38 | R1.1 11.37,206.06 11.68,205.75 | U2.2 16.25,172.88 17.25,173.88 17.25,180.62 11.75,186.12 11.75,201.38
N$5
  Top 0.61: R1.2 6.12,209.03 RV1.E
N$6
  Top 0.5: U11.6 18.88,277 20.88,275 25,275 27.75,272.25 27.75,268.75 30.12,266.38 30.12,265.53 U12.2
  Bottom 0.5: U12.15 U12.2 31,264.66 31,266 33.62,268.62 53,268.62 54.48,267.15 U13.2 U13.15
N$7
  Top 0.506: R4.1 64.21,213.46 63.62,212.88 45.69,212.88 U7.2
N$8
  Top 0.506: R5.1 64.3,210.92 63.62,210.25 47.62,210.25 46.5,209.12 44.48,209.12 U7.3
N$9
  Top 0.506: R6.1 62.88,208.38 62.25,207.75 48.88,207.75 47.62,206.5 44.4,206.5 U7.4
N$10
  Top 0.506: R7.1 62.22,205.84 61.62,205.25 49.62,205.25 48.38,204 44.44,204 U7.5
N$11
  Top 0.506: R8.1 61.92,203.3 61.38,202.75 61.25,202.75 61.12,202.62 51.12,202.62 49.75,201.25 44.52,201.25 U7.6
N$12
  Top 0.5: 46.25,198.88 55.62,198.88 56.88,200.12
  Top 0.506: R9.1 62.13,200.76 61.5,200.12 56.88,200.12 | 46.25,198.88 44.39,198.88 U7.7
N$13
  Top 0.5: 47.38,196.38 56.75,196.38 57.88,197.5
  Top 0.506: R10.1 62.34,198.22 61.62,197.5 57.88,197.5 | U7.8 44.43,196.38 47.38,196.38
N$14
  Top 0.506: R11.1 62.68,195.68 62,195 47.12,195 46,193.88 44.47,193.88 U7.9
N$15
  Top 0.506: R12.1 62.39,193.14 61.75,192.5 47.12,192.5 45.88,191.25 44.38,191.25 U7.10
N$16
  Top 0.506: R13.1 62.48,190.6 61.88,190 46.62,190 45.5,188.88 44.55,188.88 U7.11
N$17
  Top 0.5: R14.1 65.33,188.06 63.42,186.16 U7.13
N$18
  Bottom 0.5: R15.1 66.59,186.16 64.06,188.69 U7.14
N$19
  Bottom 0.5: R16.1 58.34,183.62 57.07,184.88 57.07,189.33 58.98,191.24 U7.15
N$20
  Bottom 0.5: R17.1 58.34,181.07 55.8,183.62 55.8,191.24 58.34,193.78 U7.16
N$21
  Bottom 0.5: R18.1 58.98,178.53 54.53,182.98 54.53,193.78 57.07,196.31 U7.17
N$22
  Top 0.5: R19.1 63.42,175.36 62.15,174.09
  Top 0.506: 62.15,174.09 49.78,174.09 48.62,175.25 44.48,175.25 U8.1
N$23
  Top 0.5: R20.1 64.06,172.82 62.78,171.55 47.55,171.55 46.27,172.82 U8.2
N$24
  Top 0.5: R21.1 65.96,170.28 64.69,169.01 46.27,169.01 45.01,170.28 U8.3
N$25
  Top 0.5: R22.1 63.42,167.74 62.15,166.47
  Top 0.506: U8.4 50,167.75 51.25,166.5 62.12,166.5 62.15,166.47
N$26
  Top 0.5: R23.1 63.42,165.2 62.15,163.93
  Top 0.506: 62.15,163.93 49.82,163.93 48.5,165.25 44.42,165.25 U8.5
N$27
  Top 0.5: R24.1 63.42,162.66 62.15,161.39
  Top 0.506: 62.15,161.39 48.73,161.39 47.5,162.62 44.41,162.62 U8.6
N$28
  Top 0.5: R25.1 62.78,160.12 61.52,158.85
  Top 0.506: U8.7 46.38,160.12 47.62,158.88 61.49,158.88 61.52,158.85
N$29
  Top 0.5: R26.1 63.42,157.58 62.15,156.31 45.64,156.31 U8.8
N$30
  Top 0.5: R27.1 64.69,155.04 63.42,153.77 45.64,153.77 U8.9
N$31
  Top 0.5: R28.1 65.33,152.5 64.06,151.23 45.64,151.23 U8.10
N$32
  Top 0.5: R29.1 65.96,149.96 64.69,148.69 45.64,148.69 U8.11
N$33
  Top 0.5: R30.1 U8.13
N$34
  Bottom 0.5: R31.1 60.88,148.69 U8.14
N$35
  Bottom 0.5: R32.1 58.34,145.51 57.07,146.78 57.07,151.23 58.34,152.5 U8.15
N$36
  Bottom 0.5: R33.1 58.98,142.97 55.8,146.15 55.8,151.87 58.98,155.04 U8.16
N$37
  Bottom 0.5: R34.1 59.61,140.44 54.53,145.51 54.53,153.77 58.34,157.58 U8.17
N$38
  Top 0.5: R35.1 64.42,139.17 61.88,136.62 57.5,136.62 56.25,137.88 44.39,137.88 U9.1
N$39
  Top 0.5: R36.1 64.5,136.62 62,134.12 48,134.12 46.75,135.38 44.39,135.38 U9.2
N$40
  Top 0.5: R37.1 63.96,134.08 61.38,131.5 47.38,131.5 46,132.88 44.43,132.88 U9.3
N$41
  Top 0.5: R38.1 64.3,131.55 61.75,129 50.75,129 49.5,130.25 44.4,130.25 U9.4
N$42
  Top 0.5: R39.1 64.75,129 62.25,126.5 51.25,126.5 50,127.75 44.38,127.75 U9.5
N$43
  Top 0.5: R40.1 63.97,126.47 61.38,123.88 45.69,123.88 U9.6
N$44
  Top 0.5: R41.1 70.17,123.92 67.62,121.38 45.65,121.38 U9.7
N$45
  Top 0.5: R42.1 71.39,121.39 68.88,118.88 45.61,118.88 U9.8
N$46
  Top 0.5: R43.1 71.34,118.84 68.88,116.38 45.57,116.38 U9.9
N$47
  Top 0.5: R44.1 71.06,116.31 68.5,113.75 45.66,113.75 U9.10
N$48
  Top 0.5: R45.1 70.64,113.77 68.12,111.25 47.38,111.25 46.25,112.38 44.49,112.38 U9.11
N$49
  Top 0.5: U9.13 68.83,109.95 70.25,111.38 72.64,111.38 R46.1
N$50
  Bottom 0.506: R47.1 65.42,109.95 62.88,112.5 U9.14
N$51
  Bottom 0.506: R48.1 58.09,107.41 56.88,108.62 56.88,113.62 58.12,114.88 59.45,114.88 U9.15
N$52
  Bottom 0.506: R49.1 59,104.88 55.88,108 55.88,114.88 58.5,117.5 59.53,117.5 U9.16
N$53
  Bottom 0.506: R50.1 71.17,102.34 69.75,103.75 58.5,103.75 54.75,107.5 54.75,117.25 57.62,120.12 59.6,120.12 U9.17
N$54
  Top 0.5: 66.88,100.38 72.25,100.38 72.38,100.5 72.94,100.5 R51.1
  Top 0.51: 66.88,100.38 45.06,100.38 U10.1
N$55
  Top 0.5: 66.62,97.88 72.7,97.88 R52.1
  Top 0.51: 66.62,97.88 45.5,97.88 44.38,99 43.9,99 U10.2
N$56
  Top 0.5: 66.25,95.38 72.61,95.38 R53.1
  Top 0.51: 66.25,95.38 44.98,95.38 U10.3
N$57
  Top 0.5: 66.38,92.88 72.65,92.88 R54.1
  Top 0.51: 66.38,92.88 44.94,92.88 U10.4
N$58
  Top 0.5: 66.62,90.25 72.57,90.25 R55.1
  Top 0.51: 66.62,90.25 45.02,90.25 U10.5
N$59
  Top 0.5: 66,87.75 72.61,87.75 R56.1
  Top 0.51: 66,87.75 44.98,87.75 U10.6
N$60
  Top 0.5: 66.25,85.25 72.65,85.25 R57.1
  Top 0.51: 66.25,85.25 57,85.25 55.79,86.46 U10.7
N$61
  Top 0.5: 64.75,82.62 72.56,82.62 R58.1
  Top 0.506: 43.81,84 U10.8
  Top 0.51: 64.75,82.62 45.03,82.62 U10.8
N$62
  Top 0.5: 64.12,80.12 72.6,80.12 R59.1
  Top 0.51: 64.12,80.12 44.99,80.12 U10.9
N$63
  Top 0.5: 64.12,77.5 72.52,77.5 R60.1
  Top 0.506: 43.77,78.88 U10.10
  Top 0.51: 64.12,77.5 45.08,77.5 U10.10
N$64
  Top 0.5: 63.38,75 72.56,75 R61.1
  Top 0.51: 63.38,75 45.03,75 U10.11
N$65
  Top 0.5: 63.75,73.75 70.25,73.75 71.12,72.88 72.72,72.88 R62.1
  Top 0.506: 63.75,73.75 58.98,73.75 U10.13
N$66
  Bottom 0.506: R63.1 59.29,76.62 U10.14
N$67
  Bottom 0.506: R64.1 72.45,74.08 69.5,71.12 57.5,71.12 55.88,72.75 55.88,77 57.5,78.62 58.76,78.62 U10.15
N$68
  Bottom 0.506: R65.1 72.41,71.54 71,70.12 57.25,70.12 54.88,72.5 54.88,78 58.26,81.38 U10.16
N$69
  Top 0.5: U12.1 33.64,263.24 35.88,261 44.38,261 46.62,263.25 46.62,264.33 U13.5
N$70
  Top 0.5: U5.2 16.75,148.88 18.12,150.25 29.07,150.25 U4.1
  Bottom 0.5: U4.1 U4.2
N$71
  Top 0.51: U5.4 19.18,143.8 20.38,145 28.94,145 U4.4 U4.5
N$72
  Bottom 0.5: U4.10 U4.9 36.3,138.67 32.25,134.62 27.62,134.62 27.25,135 16.44,135 U5.7
N$73
  Top 0.5: U5.1 11.8,151.42 D1.A
N$74  (via drill 0.7)
  Top 0.5: U7.18 59.59,198.88 57.62,198.88 56.38,197.62 40.62,197.62 v38.62,195.62
  Bottom 0.406: 33.12,148 33.12,162.25
  Bottom 0.5: U4.3 31.41,146.29 33.12,148 | v38.62,195.62 34.38,191.38 34.38,163.5 33.12,162.25
N$75  (via drill 0.7)
  Top 0.5: 47,161.38 35.5,161.38 v34.25,160.12
  Top 0.506: 47,161.38 48.25,160.12 U8.18
  Bottom 0.5: U4.6 30.67,138.67 34.25,142.25 v34.25,160.12
N$76  (via drill 0.7)
  Top 0.5: v55.5,136.62 38.3,136.62 U4.8
  Bottom 0.5: U9.18 57.97,122.66 56,124.62 56,136.12 v55.5,136.62
N$77
  Bottom 0.51: U10.18 58.09,86.46 52.25,80.62 52.25,74.62 49.38,71.75 42,71.75 40.5,73.25 40.5,141.06 U4.11
N$78
  Top 0.5: U5.14 19.46,146.34 18.12,145 12.12,145 11.44,144.31 D1.C
  Bottom 0.406: 32.38,163 32.38,157.75
  Bottom 0.5: U6.6 32.23,201.4 33.38,200.25 33.38,164 32.38,163 | 32.38,157.75 26.62,152 26.62,150.08 U5.14
N$79
  Bottom 0.5: U5.10 25.43,136.18 26.62,137.38 32.88,137.38 35.38,139.88 35.38,144.62 36.88,146.12 37.65,146.12 U4.12
  Bottom 0.51: U4.13 U4.12
N$80
  Top 0.61: U2.1 14.66,181.22 9.75,186.12 9.75,196.88 2.5,204.12 2.5,219.12 11.75,228.38 12,288.25 15.5,291.75 35.75,291.75 61.09,266.41 SW1.1
N$81
  Bottom 0.5: R2.2 17.91,251.28 18.62,252 18.62,256.72 U12.10
N$82
  Bottom 0.5: U12.12 23.48,249.6 R67.2
N$83
  Bottom 0.5: R68.2 21.88,235.88 25.5,239.5 25.5,244.38 26,244.88 26,256.92 U12.13
N$84
  Bottom 0.5: R69.2 15.04,241.71 13.38,243.38 13.38,254.46 U12.9
N$85
  Bottom 0.5: R70.2 18.46,235.72 22.75,240 22.75,240.12 22.88,240.25 22.88,244.62 22.25,245.25 22.25,250.5 20.94,251.81 U12.11
N$86
  Bottom 0.5: U12.6 20.88,264.5 20.88,263.75 17.25,260.12 17.25,260 17.12,259.88 17.12,252.12 15.38,250.38 15.38,249.88 15.75,249.5 15.63,249.5 R71.2
N$87
  Bottom 0.5: R72.2 20.43,250.94 19.75,251.62 19.75,260.25 22.25,262.75 22.25,266.38 21.62,267 19.5,267 18.38,265.88 18.38,264.59 U12.7
N$88
  Bottom 0.5: R73.2 34.98,249.35 41.62,256 41.62,256.79 U13.10
N$89
  Bottom 0.5: U13.12 46.85,258.39 45.62,259.62 44,259.62 43.12,258.75 43.12,258.62 43,258.62 43,253.86 R74.2
N$90
  Bottom 0.5: R75.2 43.88,233.63 49.5,239.25 49.5,256.84 U13.13
N$91
  Bottom 0.5: U13.9 33,250.71 33,239.12 29.38,235.5 29.38,233.94 R76.2
N$92
  Bottom 0.5: U13.11 44.31,239.69 43.12,238.5 43.12,238.38 33.5,238.38 31,235.88 31,232.62 30.62,232.25 28.25,232.25 26.75,233.75 R77.2
N$93
  Bottom 0.5: U13.6 44,264.88 44,266.38 42.88,267.5 33.62,267.5 32.25,266.12 32.25,252.12 31.07,250.94 R78.2
N$94
  Bottom 0.5: R79.2 32.38,233.99 32.38,234.12 33.75,235.5 42.12,235.5 48,241.38 48,259.62 45.88,261.75 42.5,261.75 41.5,262.75 41.5,264.28 U13.7
N$95
  Bottom 1.016: D68.A 30.55,284.04 27,280.5 21.75,280.5 20.5,281.75 20.5,284.94 SW3.2
N$109
  Top 0.5: 148.5,280.38 R80.2 156.33,290.91 U14.2 159.96,294.25 162.25,294.25 164.65,291.86 U14.6
  Top 0.61: 148.5,280.38 D34.A
  Top 0.813: D2.A D3.A 135.19,274.85 D4.A 135.32,272.01 D5.A D6.A 135.19,266.68 D7.A 135.07,264.07 D8.A | D17.A 135.56,204.62 D16.A 135.44,207.25 D15.A D14.A D13.A 135.31,215.25 D12.A D11.A 135.31,223 D10.A | 135.81,154.25 D18.A 135.69,151.62 D19.A 135.81,149 D20.A 135.94,146.38 D21.A 136.06,143.62 D22.A D23.A 136.19,138.25 D24.A D25.A | D26.A 136.56,77.36 D27.A 136.45,74.98 D28.A 136.69,72.25 D29.A D30.A 136.56,66.88 D31.A 136.69,64.25 D32.A 136.56,61.37 D33.A | D34.A 148.31,280.19 D35.A D36.A 148.31,272 D37.A D38.A D39.A D40.A | D49.A 149.31,204.62 D48.A D47.A 149.19,209.88 D46.A 149.31,212.62 D45.A 149.06,215.38 D44.A D43.A D42.A | D51.A 149.94,151.38 D52.A 149.94,146.38 D53.A D54.A D55.A D56.A D57.A | D58.A 150.31,77.5 D59.A 150.44,74.88 D60.A 150.31,72.12 D61.A 150.31,71.88 D62.A 150.31,66.62 D63.A 150.44,63.97 D64.A 150.57,61.21 D65.A
  Top 1.016: D8.A 135.07,263.82 D9.A 134.94,260.84 134.94,223.62 D10.A | D41.A 148.69,263.62 D40.A | 135.81,154.25 135.81,157 | 135.81,157 135.81,201.12 | 135.81,201.12 135.81,204.12 D17.A | 135.81,157 135.94,156.88 145.5,156.88 148.25,154.12 D50.A D51.A | D57.A 150.06,83.25 | 150.06,83.25 150.06,80.12 D58.A | D28.A 136.69,82.31 137.5,83.12 149.94,83.12 150.06,83.25 | 149.31,204.62 149.31,202.31 148.25,201.25 135.94,201.25 135.81,201.12
  Bottom 0.61: 135.14,280.38 D2.A
  Bottom 0.813: D34.A 148.45,280.43 147.12,281.75 147,281.75 146.62,282.12 136.89,282.12 D2.A
N$110
  Bottom 0.5: R81.2 RV3.E
N$111
  Bottom 0.5: R82.2 RV2.E
N$112
  Bottom 0.5: RV2.S 157,291.62 158,290.62 165.25,290.62 166.5,289.38 167.38,289.38 U14.5
N$113
  Bottom 0.5: RV3.S 148.5,291.62 149.75,292.88 158.79,292.88 U14.3
N$114
  Bottom 0.61: R83.1 139,295.61 D66.K
N$115
  Bottom 0.61: R84.1 131.88,295.73 D67.K
N$116
  Bottom 0.5: 120.75,288.5 131.88,288.5 132,288.38 132,288.62 | 132,288.62 132,289.95 R84.2 | U14.7 168.23,294.39 170.12,292.5 170.12,288.62 169,287.5 133.12,287.5 132,288.62
  Bottom 0.61: U17.5 119.42,289.84 120.75,288.5
N$117
  Bottom 0.5: U17.4 120.62,292.38 121.88,291.12 129.38,291.12 129.75,291.5 136.5,291.5 137.75,290.25 138.95,290.25 R83.2 139.45,290.2 142.12,292.88 147.75,292.88 149.12,294.25 149.12,296.38 151.12,298.38 158.38,298.38 U14.1
N$118
  Bottom 1.016: D68.C 60.23,284.88 C6.+ | U16.IN 62.88,278.62 60.75,280.75 60.75,283.75 60.25,284.25 60.26,284.25 C6.+ | C2.1 62.33,286.31 C6.+
N$119
  Bottom 1.016: X1.1 9.53,288.27 13.25,292 21,292 24,289 24,285.45 SW3.3
ON
  Top 0.61: SW1.3 80.66,282.28 87.62,289.25 104.75,289.25 106.75,287.25 117.77,287.25 U17.6
U7.1
  Top 0.5: U11.4 23.96,278.34 26.25,280.62 43.75,280.62 61.12,263.25 61.12,254.12 58.62,251.62 58.38,216
  Top 0.61: R3.1 58.38,216 46.27,216 U7.1
U10.17  (via drill 0.7)
  Top 0.5: v40.88,213.62 40.88,216.12 44.12,219.38 44.25,219.38 56.38,231.5 56.38,252.38 58.75,254.75 58.75,260 55.75,263 55.75,266.88 45.38,277.25 31.84,277.25 U11.1
  Top 0.51: U10.17 47.08,83.92 v45.88,85.12
  Bottom 0.5: 35.5,189.75 40.88,195.38 v40.88,213.62
  Bottom 0.506: R66.1 57,69 | 53.62,73.38 53.62,79.5
  Bottom 0.51: 35.5,189.75 35.5,151 36.38,150.12 40,150.12 41.5,148.62 41.5,85.38 41.75,85.12 v45.88,85.12 | 57,69 56.62,69 53.62,72 53.62,73.38 | 53.62,79.5 53.62,80.17 57.38,83.92 U10.17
